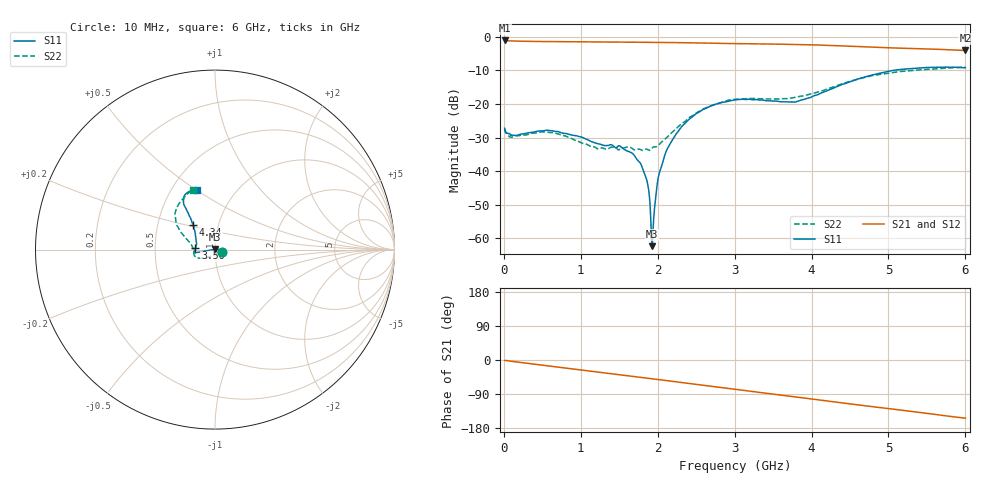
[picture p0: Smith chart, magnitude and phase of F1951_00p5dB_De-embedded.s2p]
! Integrated Device Technology
! Corporate Headquarters
! 6024 Silver Creek Valley Road
! San Jose, CA 95138  USA
! Phone:  1-408-284-8200
! Toll Free:  1-800-223-1366
! Webpage:  http://www.idt.com/
! Timing and RF Division
! 515 Groton Road, Suite 102
! Westford, MA 01886-6024
! Device:  F1951
! Description: 6-bit 0.5 dB Digital Step Attenuator
! Frequency:  100.0 -  4000.00 MHz
! Package:  4x4 mm Thin QFN Plastic Package: 24 pin
! Ports:  2 RF, 6 DC
!  Pin  1  = NC
!  Pin  2  = RF1  =  Port 1
!  Pin  3  = GND
!  Pin  4  = NC
!  Pin  5  = Serial Data Out (SDO)
!  Pin  6  = NC
!  Pin  7  = Reset Bar ( RSTb)
!  Pin  8  = Clock (CLK)
!  Pin  9  = Chip Select Bar (CSb)
!  Pin 10  = NC
!  Pin 11  = Serial Data In (SDI)
!  Pin 12  = NC
!  Pin 13  = NC
!  Pin 14  = VDD
!  Pin 15  = NC
!  Pin 16  = GND
!  Pin 17  = RF2  =  Port 2
!  Pin 18  = NC
!  Pin 19  = GND
!  Pin 20  = GND
!  Pin 21  = GND
!  Pin 22  = GND
!  Pin 23  = GND
!  Pin 24  = GND
! State:  1
! Atten State:  0.5 dB
! Voltage:  +3.30 Volts
! Current:  0.489 mA
! Data:  The device was measured on a F195X evaluation board which has
!  individual transmission lines to the RF pins.  Data was collected
!  de-embedded using a Automatic Fixture Removal [AFR] (Keysight Technologies).
!  The reference plane is the edge of the package pin.
! Misc:  Lot Code  1225BCA
!  Action Tracker AT0399
! Date Measured:  2018-09-13
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# GHz S dB R 50
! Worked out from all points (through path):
!   600 points, 10 MHz to 6 GHz, reference 50 ohm
!   highest |S21| = -1.06 dB at 10 MHz (marker M1); lowest = -4.0 dB at 6 GHz (marker M2)
!   group delay of S21, straight-line fit = 70.9 ps
!   lowest |S11| = -62.4 dB at 1.93 GHz (marker M3), VSWR 1.00, Z = 50 + j0.0696 ohm
!   |S11| at or under -10 dB: start of sweep to 5.058 GHz
!   |S22| runs from -33.8 to -9.0 dB; largest |S21 - S12| = 0.001
!   S11 on the Smith chart (normalised r, x): 10 MHz: 1.09, -0.03; 3.56 GHz: 0.80, +0.01; 4.34 GHz: 0.76, +0.21; 6 GHz: 0.67, +0.50
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0.01  -27.23 -19.2  -1.06 -1.1  -1.06 -1.1  -27.50 -21.9
0.1  -29.27 -35.4  -1.21 -3.4  -1.21 -3.4  -29.91 -36.2
0.65  -28.09 -68.9  -1.41 -17.3  -1.41 -17.3  -28.60 -76.2
1.01  -29.86 -50.0  -1.48 -26.3  -1.48 -26.3  -31.61 -60.9
1.69  -35.16 8.0  -1.57 -43.4  -1.58 -43.4  -33.61 -24.8
1.78  -37.89 10.9  -1.59 -45.7  -1.59 -45.7  -33.66 -35.9
1.85  -42.13 7.9  -1.61 -47.5  -1.61 -47.5  -33.43 -49.4
1.88  -45.24 11.1  -1.62 -48.3  -1.62 -48.3  -33.73 -54.1
1.91  -54.29 18.6  -1.63 -49.0  -1.63 -49.0  -33.65 -61.9
1.93  -62.40 113.4  -1.63 -49.6  -1.63 -49.6  -33.14 -67.8
1.95  -53.60 149.1  -1.63 -50.1  -1.63 -50.1  -32.78 -72.1
1.98  -46.48 170.7  -1.64 -50.9  -1.64 -50.9  -32.77 -77.7
2.01  -41.68 -178.1  -1.64 -51.6  -1.65 -51.6  -32.35 -85.4
2.13  -33.16 -173.5  -1.67 -54.7  -1.68 -54.8  -29.76 -106.8
2.34  -26.10 -170.9  -1.74 -60.3  -1.74 -60.3  -25.45 -130.3
2.61  -21.46 -171.1  -1.84 -67.3  -1.84 -67.3  -21.32 -145.5
3.01  -18.75 -170.9  -1.99 -77.4  -2.00 -77.4  -18.61 -160.9
3.56  -19.19 175.9  -2.16 -91.5  -2.16 -91.5  -18.57 -178.3
4.01  -17.81 146.2  -2.37 -103.2  -2.37 -103.2  -16.95 165.7
4.34  -14.75 132.0  -2.62 -111.8  -2.62 -111.8  -14.45 156.3
5.01  -10.23 124.5  -3.26 -128.5  -3.26 -128.5  -10.84 140.3
6  -9.20 106.8  -4.04 -153.5  -4.04 -153.5  -9.04 110.3
